| IBIS file stm32u073_083_lqfp80.ibs
[IBIS ver] 4.2
[File name] stm32u073_083_lqfp80.ibs
[File Rev] 0.3
[Date] 20-02-2024
[Source] Data Created at STMicroelectronics
[Notes]  File originated from ELDO simulations.
[Disclaimer]  This information is for modeling purpose only and is
   not guaranteed. The information is subject to change without
   notice.
[Copyright] Copyright 2024 STMicroelectronics Inc.
|   Component stm32u073_083_lqfp80
[Component] stm32u073_083_lqfp80
[Manufacturer] STMicroelectronics
[Package]
| variable   typ   min   max
R_pkg  0  NA  NA
L_pkg  0  NA  NA
C_pkg  0  NA  NA
[Pin]   signal_name   model_name
1  VSS  gnd
2  VDD  power
3  VBAT  power
4  PC13  io8_ft_v33
5  PC14-OSC32_IN  io8_ft_v33
6  PC15-OSC32_OUT  io8_ft
7  PF0-OSC_IN  io8_ft
8  PF1-OSC_OUT  io8_ft
9  PF2-NRST  ioreset_ft_v33
10  PC0  io8_ft_i2c
11  PC1  io8_ft_i2c
12  PC2  io8_ft
13  PC3  io8_ft
14  VSSA_VREFM  nc
15  VREFP  nc
16  VDDA  nc
17  PA0  io8_ft_v33
18  PA1  io8_ft_v33
19  PA2  io8_ft_v33
20  PA3  io8_ft
21  VSS  gnd
22  VDD  power
23  PA4  io8_ft
24  PA5  io8_ft
25  PA6  io8_ft_i2c
26  PA7  io8_ft_i2c
27  PC4  io8_ft
28  PC5  io8_ft_v33
29  PB0  io8_ft
30  PB1  io8_ft
31  PB2  io8_ft
32  PE7  io8_ft
33  PE8  io8_ft
34  PE9  io8_ft
35  PB10  io8_ft_i2c
36  PB11  io8_ft_i2c
37  VSS  gnd
38  VDD  power
39  PB12  io8_ft
40  PB13  io8_ft_i2c
41  PB14  io8_ft_i2c
42  PB15  io8_ft_v33
43  PD8  io8_ft
44  PD9  io8_ft
45  PD10  io8_ft
46  PD11  io8_ft
47  PD12  io8_ft_i2c
48  PD13  io8_ft_i2c
49  PC6  io8_ft
50  PC7  io8_ft
51  PC8  io8_ft
52  PC9  io8_ft
53  PA8  io8_ft
54  PA9  io8_ft_i2c
55  PA10  io8_ft_i2c
56  PA11  io8usb_ft_phy
57  PA12  io8usb_ft_phy
58  PA13  io8_ft
59  VSS  gnd
60  VDDUSB  power
61  PA14  io8_ft
62  PA15  io8_ft
63  PC10  io8_ft
64  PC11  io8_ft
65  PC12  io8_ft
66  PD0  io8_ft
67  PD1  io8_ft
68  PD2  io8_ft
69  PD3  io8_ft
70  PD4  io8_ft
71  PD5  io8_ft
72  PD6  io8_ft
73  PB3  io8_ft_i2c
74  PB4  io8_ft_i2c
75  PB5  io8_ft
76  PB6  io8_ft_i2c
77  PB7  io8_ft_i2c
78  PF3-BOOT0  io8_ft_v33
79  PB8  io8_ft_i2c
80  PB9  io8_ft_i2c
[Package Model]   489-lqfp-12x12-80-ldo-250125
[Pin Mapping]   pulldown_ref   pullup_ref   | Comment
1  gndio  nc
2  nc  vddio
3  nc  vsw
4  gndio  vddio  | Depending on IO usage
| 4  gndio  vsw  | Depending on IO usage
5  gndio  vddio  | Depending on IO usage
| 5  gndio  vsw  | Depending on IO usage
6  gndio  vddio  | Depending on IO usage
| 6  gndio  vsw  | Depending on IO usage
7  gndio  vddio
8  gndio  vddio
9  gndio  vddio
10  gndio  vddio
11  gndio  vddio
12  gndio  vddio
13  gndio  vddio
14  nc  nc
15  nc  nc
16  nc  nc
17  gndio  vddio
18  gndio  vddio
19  gndio  vddio
20  gndio  vddio
21  gndio  nc
22  nc  vddio
23  gndio  vddio
24  gndio  vddio
25  gndio  vddio
26  gndio  vddio
27  gndio  vddio
28  gndio  vddio
29  gndio  vddio
30  gndio  vddio
31  gndio  vddio
32  gndio  vddio
33  gndio  vddio
34  gndio  vddio
35  gndio  vddio
36  gndio  vddio
37  gndio  nc
38  nc  vddio
39  gndio  vddio
40  gndio  vddio
41  gndio  vddio
42  gndio  vddio
43  gndio  vddio
44  gndio  vddio
45  gndio  vddio
46  gndio  vddio
47  gndio  vddio
48  gndio  vddio
49  gndio  vddio
50  gndio  vddio
51  gndio  vddio
52  gndio  vddio
53  gndio  vddio
54  gndio  vddio
55  gndio  vddio
56  gndio  vddusb  | Depending on IO usage
| 56  gndio  vddio  | Depending on IO usage
57  gndio  vddusb  | Depending on IO usage
| 57  gndio  vddio  | Depending on IO usage
58  gndio  vddio
59  gndio  nc
60  nc  vddusb
61  gndio  vddio
62  gndio  vddio
63  gndio  vddio
64  gndio  vddio
65  gndio  vddio
66  gndio  vddio
67  gndio  vddio
68  gndio  vddio
69  gndio  vddio
70  gndio  vddio
71  gndio  vddio
72  gndio  vddio
73  gndio  vddio
74  gndio  vddio
75  gndio  vddio
76  gndio  vddio
77  gndio  vddio
78  gndio  vddio
79  gndio  vddio
80  gndio  vddio
|[Diff Pin]  inv_pin  vdiff  tdelay_typ  tdelay_min  tdelay_max
|57  56  NA  NA  NA  NA
[Model Selector] io8_ft
io8_ft_ls_1v2   "GPIO - 5V tolerant - 1.2V range - Low speed"
io8_ft_ms_1v2   "GPIO - 5V tolerant - 1.2V range - Med speed"
io8_ft_fs_1v2   "GPIO - 5V tolerant - 1.2V range - Fast speed"
io8_ft_hs_1v2   "GPIO - 5V tolerant - 1.2V range - High speed"
io8_ft_ls_1v8   "GPIO - 5V tolerant - 1.8V range - Low speed"
io8_ft_ms_1v8   "GPIO - 5V tolerant - 1.8V range - Med speed"
io8_ft_fs_1v8   "GPIO - 5V tolerant - 1.8V range - Fast speed"
io8_ft_hs_1v8   "GPIO - 5V tolerant - 1.8V range - High speed"
io8_ft_ls_3v3   "GPIO - 5V tolerant - 3.3V range - Low speed"
io8_ft_ms_3v3   "GPIO - 5V tolerant - 3.3V range - Med speed"
io8_ft_fs_3v3   "GPIO - 5V tolerant - 3.3V range - Fast speed"
io8_ft_hs_3v3   "GPIO - 5V tolerant - 3.3V range - High speed"
[Model Selector] io8_ft_i2c
io8_ft_ls_1v2   "GPIO - 5V tolerant - 1.2V range - Low speed"
io8_ft_ms_1v2   "GPIO - 5V tolerant - 1.2V range - Med speed"
io8_ft_fs_1v2   "GPIO - 5V tolerant - 1.2V range - Fast speed"
io8_ft_hs_1v2   "GPIO - 5V tolerant - 1.2V range - High speed"
io8_ft_ls_1v8   "GPIO - 5V tolerant - 1.8V range - Low speed"
io8_ft_ms_1v8   "GPIO - 5V tolerant - 1.8V range - Med speed"
io8_ft_fs_1v8   "GPIO - 5V tolerant - 1.8V range - Fast speed"
io8_ft_hs_1v8   "GPIO - 5V tolerant - 1.8V range - High speed"
io8_ft_ls_3v3   "GPIO - 5V tolerant - 3.3V range - Low speed"
io8_ft_ms_3v3   "GPIO - 5V tolerant - 3.3V range - Med speed"
io8_ft_fs_3v3   "GPIO - 5V tolerant - 3.3V range - Fast speed"
io8_ft_hs_3v3   "GPIO - 5V tolerant - 3.3V range - High speed"
io8_ft_i2c_ls_1v2   "GPIO I2C open-drain - 5V tolerant - 1.2V range - Low speed"
io8_ft_i2c_ms_1v2   "GPIO I2C open-drain - 5V tolerant - 1.2V range - Med speed"
io8_ft_i2c_fs_1v2   "GPIO I2C open-drain - 5V tolerant - 1.2V range - Fast speed"
io8_ft_i2c_hs_1v2   "GPIO I2C open-drain - 5V tolerant - 1.2V range - High speed"
io8_ft_i2c_ls_1v8   "GPIO I2C open-drain - 5V tolerant - 1.8V range - Low speed"
io8_ft_i2c_ms_1v8   "GPIO I2C open-drain - 5V tolerant - 1.8V range - Med speed"
io8_ft_i2c_fs_1v8   "GPIO I2C open-drain - 5V tolerant - 1.8V range - Fast speed"
io8_ft_i2c_hs_1v8   "GPIO I2C open-drain - 5V tolerant - 1.8V range - High speed"
io8_ft_i2c_ls_3v3   "GPIO I2C open-drain - 5V tolerant - 3.3V range - Low speed"
io8_ft_i2c_ms_3v3   "GPIO I2C open-drain - 5V tolerant - 3.3V range - Med speed"
io8_ft_i2c_fs_3v3   "GPIO I2C open-drain - 5V tolerant - 3.3V range - Fast speed"
io8_ft_i2c_hs_3v3   "GPIO I2C open-drain - 5V tolerant - 3.3V range - High speed"
io8_ft_i2c_fmp_3v3   "GPIO I2C open-drain fm+ - 5V tolerant - 3.3V range"
[Model Selector] io8_ft_v33
io8_ft_v33_ls_1v2   "GPIO_V33 - 5V tolerant - 1.2V range - Low speed"
io8_ft_v33_ms_1v2   "GPIO_V33 - 5V tolerant - 1.2V range - Med speed"
io8_ft_v33_fs_1v2   "GPIO_V33 - 5V tolerant - 1.2V range - Fast speed"
io8_ft_v33_hs_1v2   "GPIO_V33 - 5V tolerant - 1.2V range - High speed"
io8_ft_v33_ls_1v8   "GPIO_V33 - 5V tolerant - 1.8V range - Low speed"
io8_ft_v33_ms_1v8   "GPIO_V33 - 5V tolerant - 1.8V range - Med speed"
io8_ft_v33_fs_1v8   "GPIO_V33 - 5V tolerant - 1.8V range - Fast speed"
io8_ft_v33_hs_1v8   "GPIO_V33 - 5V tolerant - 1.8V range - High speed"
io8_ft_v33_ls_3v3   "GPIO_V33 - 5V tolerant - 3.3V range - Low speed"
io8_ft_v33_ms_3v3   "GPIO_V33 - 5V tolerant - 3.3V range - Med speed"
io8_ft_v33_fs_3v3   "GPIO_V33 - 5V tolerant - 3.3V range - Fast speed"
io8_ft_v33_hs_3v3   "GPIO_V33 - 5V tolerant - 3.3V range - High speed"
[Model Selector] io8usb_ft_phy
io8_ft_ls_1v2   "GPIO - 5V tolerant - 1.2V range - Low speed"
io8_ft_ms_1v2   "GPIO - 5V tolerant - 1.2V range - Med speed"
io8_ft_fs_1v2   "GPIO - 5V tolerant - 1.2V range - Fast speed"
io8_ft_hs_1v2   "GPIO - 5V tolerant - 1.2V range - High speed"
io8_ft_ls_1v8   "GPIO - 5V tolerant - 1.8V range - Low speed"
io8_ft_ms_1v8   "GPIO - 5V tolerant - 1.8V range - Med speed"
io8_ft_fs_1v8   "GPIO - 5V tolerant - 1.8V range - Fast speed"
io8_ft_hs_1v8   "GPIO - 5V tolerant - 1.8V range - High speed"
io8_ft_ls_3v3   "GPIO - 5V tolerant - 3.3V range - Low speed"
io8_ft_ms_3v3   "GPIO - 5V tolerant - 3.3V range - Med speed"
io8_ft_fs_3v3   "GPIO - 5V tolerant - 3.3V range - Fast speed"
io8_ft_hs_3v3   "GPIO - 5V tolerant - 3.3V range - High speed"
io8usb_ft_phy_hs_3v3   "USB full speed"
io8usb_ft_phy_ls_3v3   "USB low speed"
[Model Selector] ioreset_ft_v33
ioreset_ft_v33_1v2   "Reset PAD. 5V tolerant. 1.2V range"
ioreset_ft_v33_1v8   "Reset PAD. 5V tolerant. 1.8V range"
ioreset_ft_v33_3v3   "Reset PAD. 5V tolerant. 3.3V range"
[Define Package Model]  489-lqfp-12x12-80-ldo-250125
[Manufacturer]  Unknown
[OEM]  Unknown
[Description]  None
[Number Of Pins]  77
[Pin Numbers]
| Pin Num   Terminal Name
17 | PA0
18 | PA1
19 | PA2
20 | PA3
23 | PA4
24 | PA5
25 | PA6
26 | PA7
53 | PA8
54 | PA9
55 | PA10
56 | PA11
57 | PA12
58 | PA13
61 | PA14
62 | PA15
29 | PB0
30 | PB1
31 | PB2
73 | PB3
74 | PB4
75 | PB5
76 | PB6
77 | PB7
79 | PB8
80 | PB9
35 | PB10
36 | PB11
39 | PB12
40 | PB13
41 | PB14
42 | PB15
10 | PC0
11 | PC1
12 | PC2
13 | PC3
27 | PC4
28 | PC5
49 | PC6
50 | PC7
51 | PC8
52 | PC9
63 | PC10
64 | PC11
65 | PC12
4 | PC13
5 | PC14-OSC32_IN
6 | PC15-OSC32_OUT
66 | PD0
67 | PD1
68 | PD2
69 | PD3
70 | PD4
71 | PD5
72 | PD6
43 | PD8
44 | PD9
45 | PD10
46 | PD11
47 | PD12
48 | PD13
32 | PE7
33 | PE8
34 | PE9
7 | PF0-OSC_IN
8 | PF1-OSC_OUT
9 | PF2-NRST
78 | PF3-BOOT0
3 | VBAT
2 | VDD
22 | VDD
38 | VDD
16 | VDDA
60 | VDDUSB
15 | VREFP
1 | VSS
14 | VREFM
|[Merged Pins]  1
|21  |  VSS
|37  |  VSS
|59  |  VSS
[Model Data]
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[End Model Data]
[End Package Model]
|End [Component]
| Models and submodels in the file (42): io8_ft_fs_1v2 (I/O), io8_ft_fs_1v8 (I/O), io8_ft_fs_3v3 (I/O), io8_ft_hs_1v2 (I/O), io8_ft_hs_1v8 (I/O), io8_ft_hs_3v3 (I/O), io8_ft_i2c_fmp_3v3 (I/O_open_drain), io8_ft_i2c_fs_1v2 (I/O_open_drain), io8_ft_i2c_fs_1v8 (I/O_open_drain), io8_ft_i2c_fs_3v3 (I/O_open_drain), io8_ft_i2c_hs_1v2 (I/O_open_drain), io8_ft_i2c_hs_1v8 (I/O_open_drain), io8_ft_i2c_hs_3v3 (I/O_open_drain), io8_ft_i2c_ls_1v2 (I/O_open_drain), io8_ft_i2c_ls_1v8 (I/O_open_drain), io8_ft_i2c_ls_3v3 (I/O_open_drain), io8_ft_i2c_ms_1v2 (I/O_open_drain), io8_ft_i2c_ms_1v8 (I/O_open_drain), io8_ft_i2c_ms_3v3 (I/O_open_drain), io8_ft_ls_1v2 (I/O), io8_ft_ls_1v8 (I/O), io8_ft_ls_3v3 (I/O), io8_ft_ms_1v2 (I/O), io8_ft_ms_1v8 (I/O), io8_ft_ms_3v3 (I/O), io8_ft_v33_fs_1v2 (I/O), io8_ft_v33_fs_1v8 (I/O), io8_ft_v33_fs_3v3 (I/O), io8_ft_v33_hs_1v2 (I/O), io8_ft_v33_hs_1v8 (I/O), io8_ft_v33_hs_3v3 (I/O), io8_ft_v33_ls_1v2 (I/O), io8_ft_v33_ls_1v8 (I/O), io8_ft_v33_ls_3v3 (I/O), io8_ft_v33_ms_1v2 (I/O), io8_ft_v33_ms_1v8 (I/O), io8_ft_v33_ms_3v3 (I/O), io8usb_ft_phy_hs_3v3 (I/O), io8usb_ft_phy_ls_3v3 (I/O), ioreset_ft_v33_1v2 (I/O_open_drain), ioreset_ft_v33_1v8 (I/O_open_drain), ioreset_ft_v33_3v3 (I/O_open_drain)
